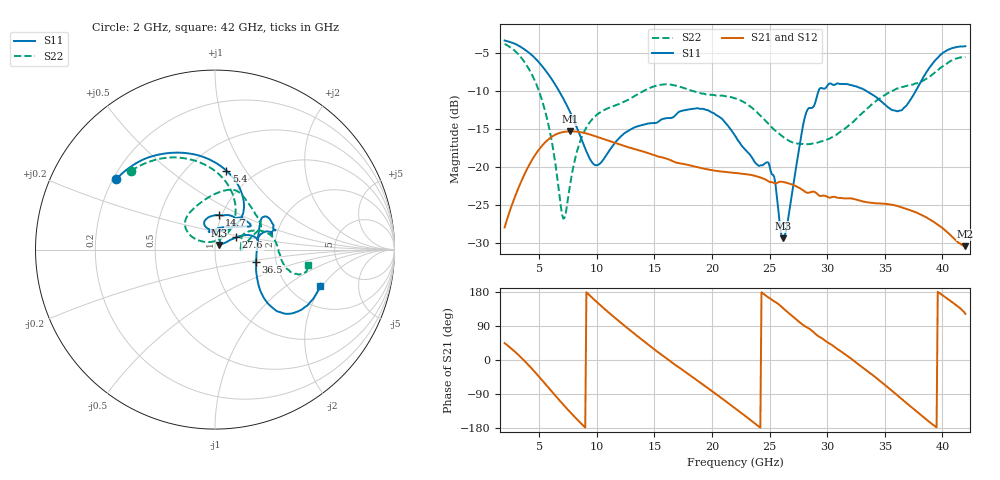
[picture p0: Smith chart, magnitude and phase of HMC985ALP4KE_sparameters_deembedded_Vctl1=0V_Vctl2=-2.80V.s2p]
!s2p File: Measurements: S11, S21, S12, S22
# GHz S dB R 50.0
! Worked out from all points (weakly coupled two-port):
!   401 points, 2 GHz to 42 GHz, reference 50 ohm
!   highest |S21| = -15.31 dB at 7.7 GHz (marker M1); lowest = -30.4 dB at 42 GHz (marker M2)
!   lowest |S11| = -29.3 dB at 26.2 GHz (marker M3), VSWR 1.07, Z = 52.3 + j2.66 ohm
!   |S11| at or under -10 dB: 6.718 GHz to 29.26 GHz (22.54 GHz wide, 125 % of centre); 33.39 GHz to 37.7 GHz (4.31 GHz wide, 12.1 % of centre)
!   |S22| runs from -26.7 to -3.9 dB; largest |S21 - S12| = 0.00071
!   S11 on the Smith chart (normalised r, x): 2 GHz: 0.21, +0.31; 5.4 GHz: 0.75, +0.82; 14.7 GHz: 0.97, +0.39; 27.6 GHz: 1.26, +0.18; 36.5 GHz: 1.57, -0.22; 42 GHz: 2.92, -1.90
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2  -3.40 144.6  -27.90 44.6  -27.88 44.6  -3.86 136.9
3.5  -4.34 118.3  -21.68 4.5  -21.69 4.5  -5.77 104.1
5.4  -7.03 81.9  -16.94 -58.5  -16.96 -58.6  -12.02 62.7
7  -10.75 56.1  -15.42 -114.6  -15.45 -114.7  -26.30 85.0
7.7  -12.82 50.3  -15.31 -137.9  -15.31 -137.9  -22.16 145.7
8.7  -16.44 52.9  -15.45 -169.3  -15.45 -169.3  -16.05 150.1
10  -19.75 86.8  -16.01 153.1  -16.00 153.1  -13.14 139.5
14.7  -14.24 83.2  -18.28 35.0  -18.25 35.0  -9.56 81.2
15.4  -13.99 74.0  -18.64 18.9  -18.65 18.8  -9.24 75.3
19.3  -12.39 33.8  -20.20 -66.5  -20.20 -66.6  -10.37 43.4
22  -15.87 52.2  -20.76 -127.2  -20.79 -127.3  -10.98 25.8
25  -19.84 99.3  -21.94 163.1  -21.90 163.1  -14.49 14.3
26.2  -29.31 48.0  -21.94 136.0  -21.99 135.9  -16.07 3.2
27.6  -17.26 30.0  -22.73 99.9  -22.74 99.8  -16.91 -3.7
28.1  -13.24 21.0  -23.24 88.7  -23.29 88.6  -17.00 -2.6
28.7  -12.22 13.0  -23.22 76.8  -23.21 76.8  -16.91 1.3
31  -9.05 23.3  -24.03 26.8  -24.02 26.8  -15.52 25.9
33.3  -9.92 34.2  -24.55 -24.7  -24.53 -24.7  -12.59 26.6
35.4  -12.27 11.9  -24.88 -75.5  -24.86 -75.5  -10.21 17.0
36.5  -12.51 -16.4  -25.28 -103.7  -25.30 -103.8  -9.49 10.3
39.5  -5.83 -43.4  -27.42 -177.8  -27.38 -177.7  -7.39 -15.4
42  -4.15 -18.9  -30.36 121.7  -30.35 121.7  -5.57 -9.4
